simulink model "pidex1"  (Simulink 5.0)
settings: Solver=ode45  StartTime=0.0  StopTime=100  MaxStep=1e-3  RelTol=1e-3

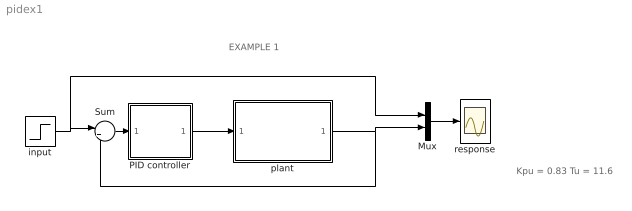
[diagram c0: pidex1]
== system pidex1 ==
  note: EXAMPLE 1
  note: Kpu = 0.83 Tu = 11.6
  Mux : Mux  Inputs=2
  PID controller : Subsystem  mask{Kp=0.5, Ki=0.09, Kd=0.77, sat=inf}
      mask prompts: Kp "Proportional gain (Kp)"; Ki "Integral gain (Ki)"; Kd "Derivative gain (Kd)"; sat "Saturation limit [pu]"
      mask help: Proportional-Integral Speed Controller
  Sum : Sum  Inputs=|+-
  input : Step  Time=.05  SampleTime=0
  plant : Subsystem
  response : Scope
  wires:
  plant/1(Out1) -> Mux/2, Sum/2
  Sum/1 -> PID controller/1(er)
  PID controller/1(c) -> plant/1(In1)
  input/1 -> Sum/1, Mux/1
  Mux/1 -> response/1

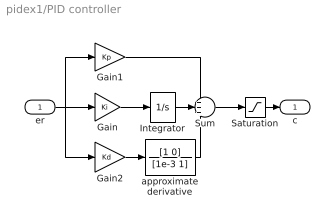
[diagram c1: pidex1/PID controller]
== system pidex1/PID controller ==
  er : Inport
  Gain : Gain  Gain=Ki
  Gain1 : Gain  Gain=Kp
  Gain2 : Gain  Gain=Kd
  Integrator : Integrator  LimitOutput=on  UpperSaturationLimit=sat  LowerSaturationLimit=-sat
  Saturation : Saturate  UpperLimit=sat  LowerLimit=-sat
  Sum : Sum  Inputs=+++
  approximate derivative : TransferFcn  Numerator=[1 0]  Denominator=[1e-3 1]
  c : Outport  InitialOutput=0
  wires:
  Gain1/1 -> Sum/1
  Gain/1 -> Integrator/1
  er/1 -> Gain/1, Gain1/1, Gain2/1
  Sum/1 -> Saturation/1
  Saturation/1 -> c/1
  Integrator/1 -> Sum/2
  Gain2/1 -> approximate derivative/1
  approximate derivative/1 -> Sum/3

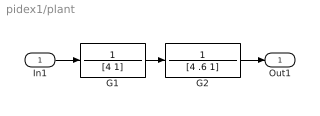
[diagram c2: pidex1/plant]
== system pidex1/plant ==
  In1 : Inport
  G1 : TransferFcn  Numerator=1  Denominator=[4 1]
  G2 : TransferFcn  Numerator=1  Denominator=[4 .6 1]
  Out1 : Outport
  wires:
  G1/1 -> G2/1
  In1/1 -> G1/1
  G2/1 -> Out1/1
